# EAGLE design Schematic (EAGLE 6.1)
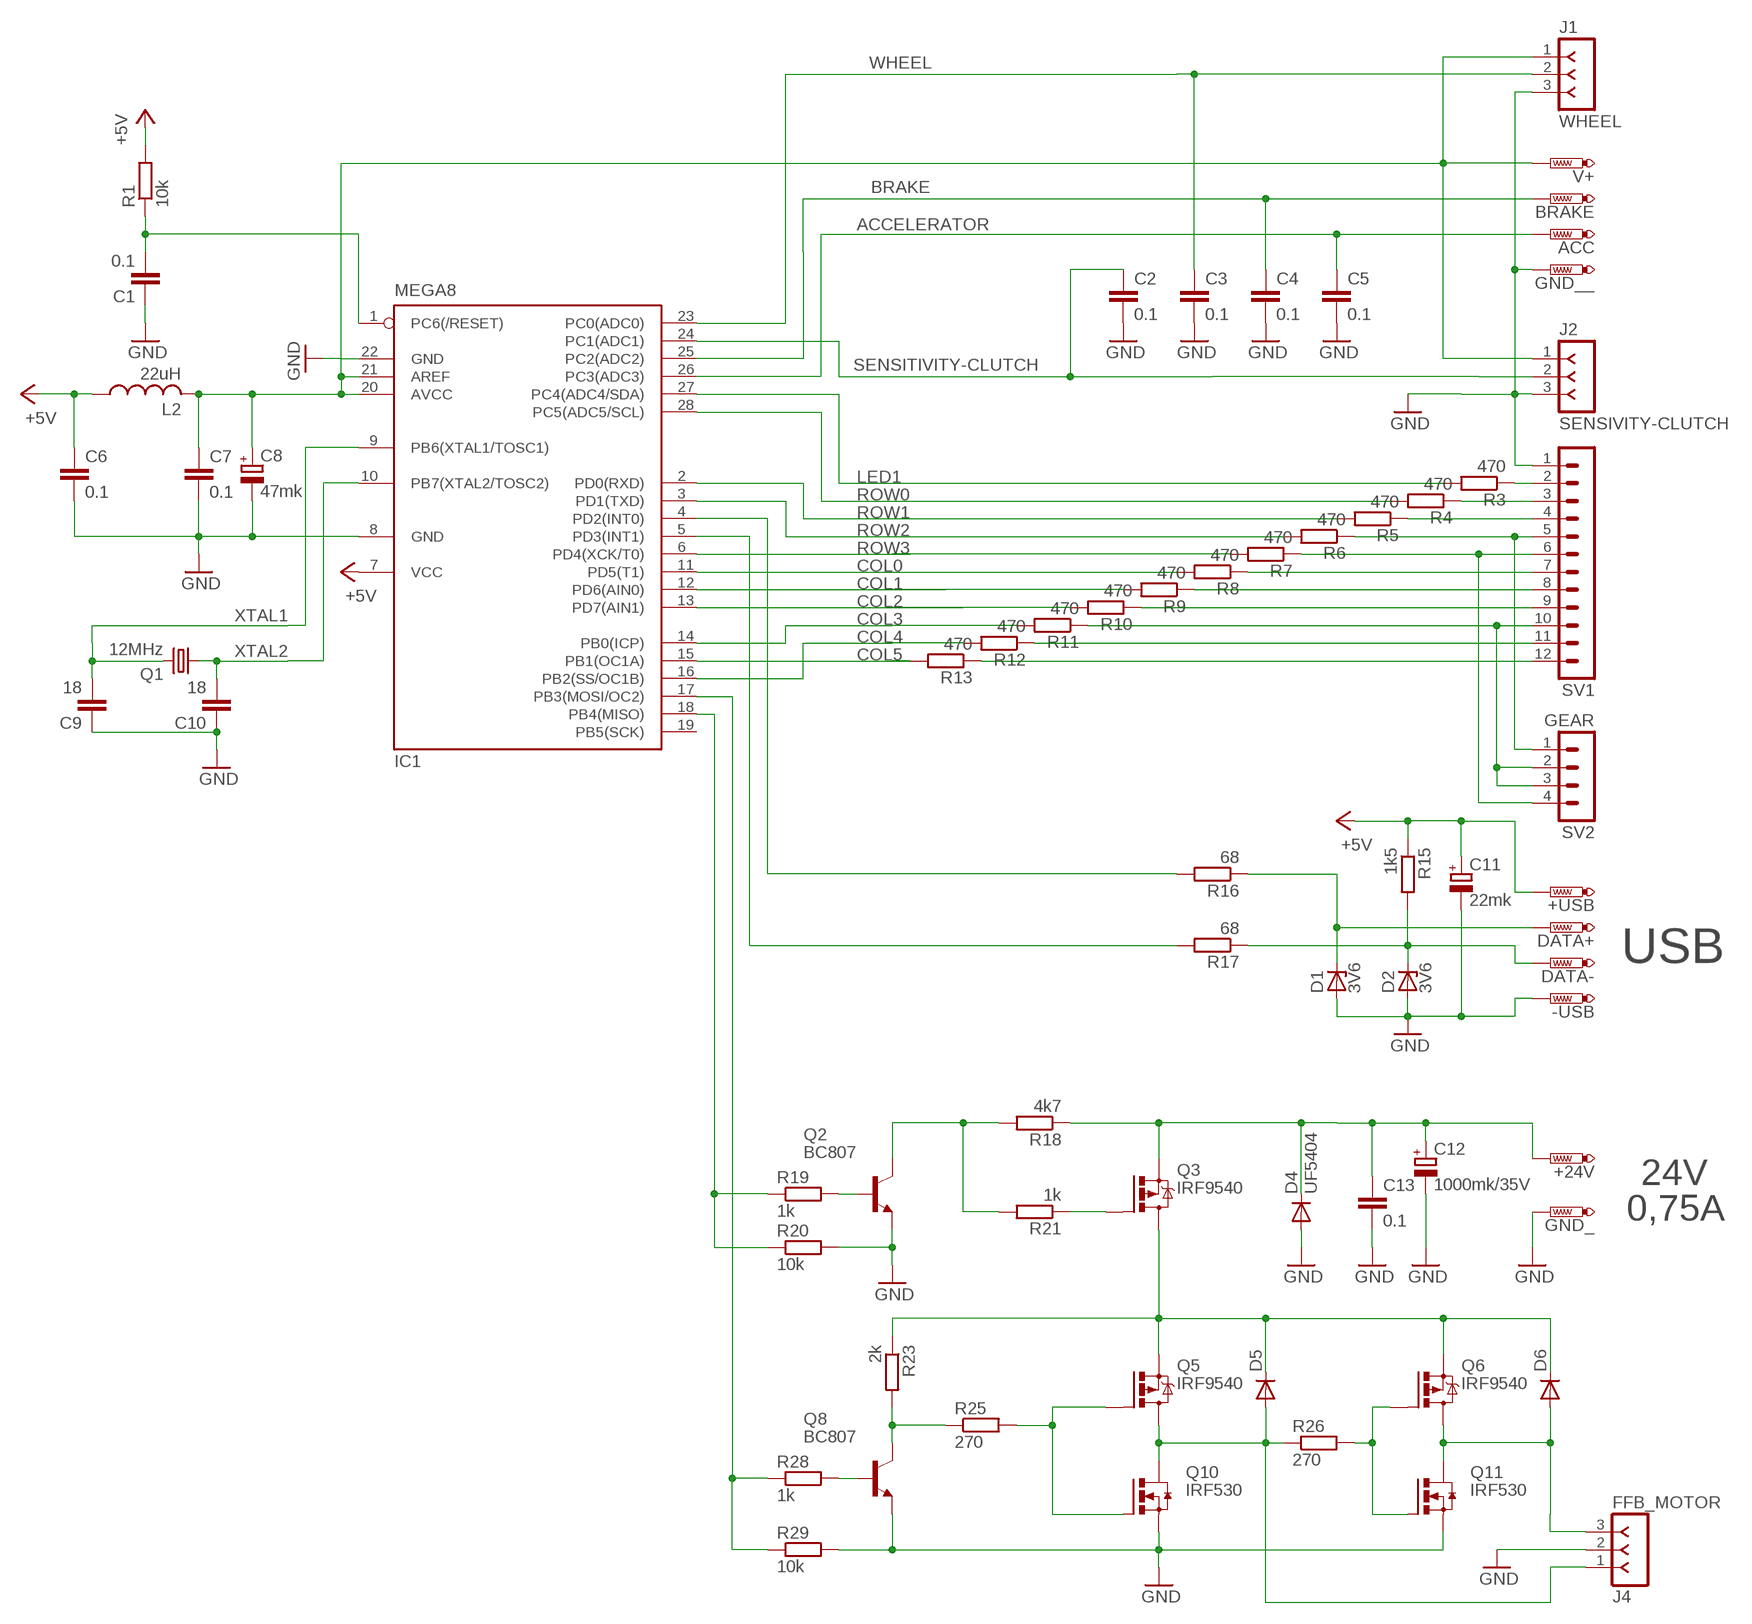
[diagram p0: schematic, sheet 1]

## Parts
+24V  PTR1PAD1-13  [P1-13]
+USB  PTR1PAD1-13  [P1-13]
-USB  PTR1PAD1-13  [P1-13]
ACC  PTR1PAD1-13  [P1-13]
BRAKE  PTR1PAD1-13  [P1-13]
C1  0.1  C-EUC0805  [C0805]
C2  0.1  C-EUC0805  [C0805]
C3  0.1  C-EUC0805  [C0805]
C4  0.1  C-EUC0805  [C0805]
C5  0.1  C-EUC0805  [C0805]
C6  0.1  C-EUC0805  [C0805]
C7  0.1  C-EUC0805  [C0805]
C8  47mk  CPOL-EUE2.5-6  [E2,5-6]
C9  18  C-EUC0805  [C0805]
C10  18  C-EUC0805  [C0805]
C11  22mk  CPOL-EUE2.5-6  [E2,5-6]
C12  1000mk/35V  CPOL-EUTT5D11L  [TT5D11L]
C13  0.1  C-EU075-032X103  [C075-032X103]
D1  3V6  BZX84CSMD  [TO236]
D2  3V6  BZX84CSMD  [TO236]
D4  UF5404  1N5400  [DO201-15]
D5  1N5400  [DO201-15]
D6  1N5400  [DO201-15]
DATA+  PTR1PAD1-13  [P1-13]
DATA-  PTR1PAD1-13  [P1-13]
GND_  PTR1PAD1-13  [P1-13]
GND__  PTR1PAD1-13  [P1-13]
IC1  MEGA8  MEGA8-P  [DIL28-3]
J1  WHEEL  F-1X03-SIP-100-32Y  [SIP-100-03-32Y]
J2  SENSIVITY-CLUTCH  F-1X03-SIP-100-32Y  [SIP-100-03-32Y]
J4  FFB_MOTOR  F-1X03-SIP-100-32Y  [SIP-100-03-32Y]
L2  22uH  L-USL3216C  [L3216C]
Q1  12MHz  CRYTALHC49U-V  [HC49U-V]
Q2  BC807  BC847SMD  [SOT23]
Q3  IRF9540  IRF4905  [TO220BH]
Q5  IRF9540  IRF4905  [TO220BH]
Q6  IRF9540  IRF4905  [TO220BH]
Q8  BC807  BC847SMD  [SOT23]
Q10  IRF530  IRFI540NPBF  [TO220BH]
Q11  IRF530  IRFI540NPBF  [TO220BH]
R1  10k  R-EU_R0805  [R0805]
R3  470  R-EU_R0805  [R0805]
R4  470  R-EU_R0805  [R0805]
R5  470  R-EU_R0805  [R0805]
R6  470  R-EU_R0805  [R0805]
R7  470  R-EU_R0805  [R0805]
R8  470  R-EU_R0805  [R0805]
R9  470  R-EU_R0805  [R0805]
R10  470  R-EU_R0805  [R0805]
R11  470  R-EU_R0805  [R0805]
R12  470  R-EU_R0805  [R0805]
R13  470  R-EU_R0805  [R0805]
R15  1k5  R-EU_R0805  [R0805]
R16  68  R-EU_0207/12  [0207/12]
R17  68  R-EU_0207/12  [0207/12]
R18  4k7  R-EU_R0805  [R0805]
R19  1k  R-EU_R0805  [R0805]
R20  10k  R-EU_R0805  [R0805]
R21  1k  R-EU_R0805  [R0805]
R23  2k  R-EU_R0805  [R0805]
R25  270  R-EU_R1206  [R1206]
R26  270  R-EU_R1206  [R1206]
R28  1k  R-EU_R0805  [R0805]
R29  10k  R-EU_R0805  [R0805]
SV1  MA12-1  [MA12-1]
SV2  GEAR  MA04-1  [MA04-1]
V+  PTR1PAD1-13  [P1-13]

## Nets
+5V: +USB.1(TP) C6.1 C11.+ IC1.7(VCC) L2.1 R1.2 R15.1
ACCELERATOR: ACC.1(TP) C5.1 IC1.26(PC3(ADC3))
BRAKE: BRAKE.1(TP) C4.1 IC1.25(PC2(ADC2))
COL0: IC1.11(PD5(T1)) R8.2
COL1: IC1.12(PD6(AIN0)) R9.2
COL2: IC1.13(PD7(AIN1)) R10.2
COL3: IC1.14(PB0(ICP)) R11.2
COL4: IC1.16(PB2(SS/OC1B)) R12.2
COL5: IC1.15(PB1(OC1A)) R13.2
FEEDBACK_MOTOR: IC1.17(PB3(MOSI/OC2)) R28.1 R29.1
GND: -USB.1(TP) C1.1 C2.2 C3.2 C4.2 C5.2 C6.2 C7.2 C8.- C9.1 C10.1 C11.- C12.- C13.2 D1.A D2.A D4.A GND_.1(TP) GND__.1(TP) IC1.8(GND) IC1.22(GND) J1.3 J2.3 J4.2 Q2.2(E) Q8.2(E) Q10.S Q11.S R20.2 R29.2 SV1.1
LED1: IC1.27(PC4(ADC4/SDA)) R3.2
M1: D5.A J4.1 Q5.D Q10.D R26.1
M2: D6.A J4.3 Q6.D Q11.D
N$1: D5.C D6.C Q3.D Q5.S Q6.S R23.1
N$2: C7.1 C8.+ IC1.20(AVCC) IC1.21(AREF) J1.1 J2.1 L2.2 V+.1(TP)
N$3: IC1.18(PB4(MISO)) R19.1 R20.1
N$4: +24V.1(TP) C12.+ C13.1 D4.C Q3.S R18.1
N$5: Q2.1(B) R19.2
N$6: IC1.5(PD3(INT1)) R17.2
N$8: IC1.4(PD2(INT0)) R16.2
N$9: D2.C DATA-.1(TP) R15.2 R17.1
N$10: D1.C DATA+.1(TP) R16.1
N$11: C1.2 IC1.1(PC6(/RESET)) R1.1
N$13: Q8.1(B) R28.2
N$14: Q8.3(C) R23.2 R25.1
N$15: R13.1 SV1.12
N$16: R11.1 SV1.10 SV2.2 SV2.3
N$19: Q5.G Q10.G R25.2
N$22: Q2.3(C) R18.2 R21.2
N$23: Q6.G Q11.G R26.2
N$30: R3.1 SV1.2
N$31: R4.1 SV1.3
N$32: R5.1 SV1.4
N$33: R6.1 SV1.5 SV2.1
N$34: R7.1 SV1.6 SV2.4
N$35: R8.1 SV1.7
N$36: R9.1 SV1.8
N$37: R10.1 SV1.9
N$39: R12.1 SV1.11
N$41: Q3.G R21.1
ROW0: IC1.28(PC5(ADC5/SCL)) R4.2
ROW1: IC1.2(PD0(RXD)) R5.2
ROW2: IC1.3(PD1(TXD)) R6.2
ROW3: IC1.6(PD4(XCK/T0)) R7.2
SENSITIVITY-CLUTCH: C2.1 IC1.24(PC1(ADC1)) J2.2
WHEEL: C3.1 IC1.23(PC0(ADC0)) J1.2
XTAL1: C9.2 IC1.9(PB6(XTAL1/TOSC1)) Q1.2
XTAL2: C10.2 IC1.10(PB7(XTAL2/TOSC2)) Q1.1
Unconnected: IC1.19(PB5(SCK))

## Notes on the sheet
- USB
- 24V
- 0,75A

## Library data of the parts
+24V +USB -USB ACC BRAKE DATA+ DATA- GND_ GND__ V+ = testpad:PTR1: TEST PIN
C1-C7 C9 C10 C13 = rcl:C-EU: CAPACITOR, European symbol
C8 C11 C12 = rcl:CPOL-EU: POLARIZED CAPACITOR, European symbol
D1 D2 = diode:BZX84CSMD: Z DIODE
D4-D6 = diode:1N5400: DIODE
IC1 = atmel:MEGA8-P: MICROCONTROLLER 8 Kbytes FLASH, 1 kbytes SRAM, 512 bytes EEPROM, USART, 4-channel 10 bit ADC, 2-channel 8 bit ADC Pin compatible with Atmega48, ATMega88, ATMega168 Source: avr.lbr; OC_FARNELL: unknown; OC_NEWARK: unknown
J1 J2 J4 = con-headers-jp:F-1X03-: FEMALE HEADER
L2 = rcl:L-US: INDUCTOR, American symbol
Q1 = crystal:CRYTAL: CRYSTAL
Q2 Q8 = transistor-npn:BC847*: NPN Transistor
Q3 Q5 Q6 = transistor-power:IRF4905: P-Channel HEXFET® Power MOSFET RDS(on)= 0.02 Ohm, ID = -74A Source: http://www.irf.com/product-info/datasheets/data/irf4905pbf.pdf
Q10 Q11 = transistor-power:IRFI540NPBF: HEXFET Power MOISFET VDSS = 100V, RDS(on) = 0.052 Ohm, ID = 20A, VGS(th) = 2.0 -- 4.0V Source: http://www.irf.com/product-info/datasheets/data/irfi540npbf.pdf
R1 R3-R13 R15-R21 R23 R25 R26 R28 R29 = rcl:R-EU_: RESISTOR, European symbol
SV1 = con-lstb:MA12-1: PIN HEADER; OC_FARNELL: unknown; OC_NEWARK: unknown
SV2 = con-lstb:MA04-1: PIN HEADER; OC_FARNELL: unknown; OC_NEWARK: unknown

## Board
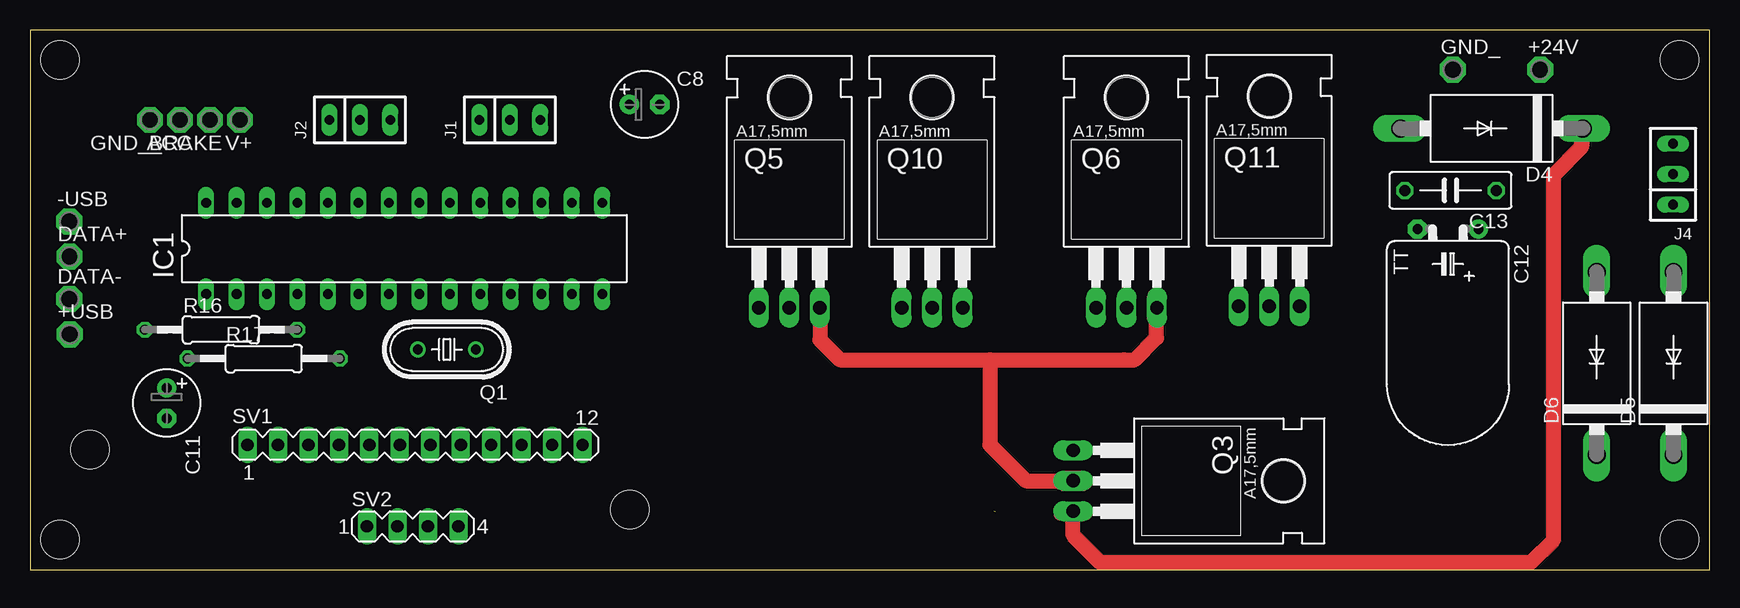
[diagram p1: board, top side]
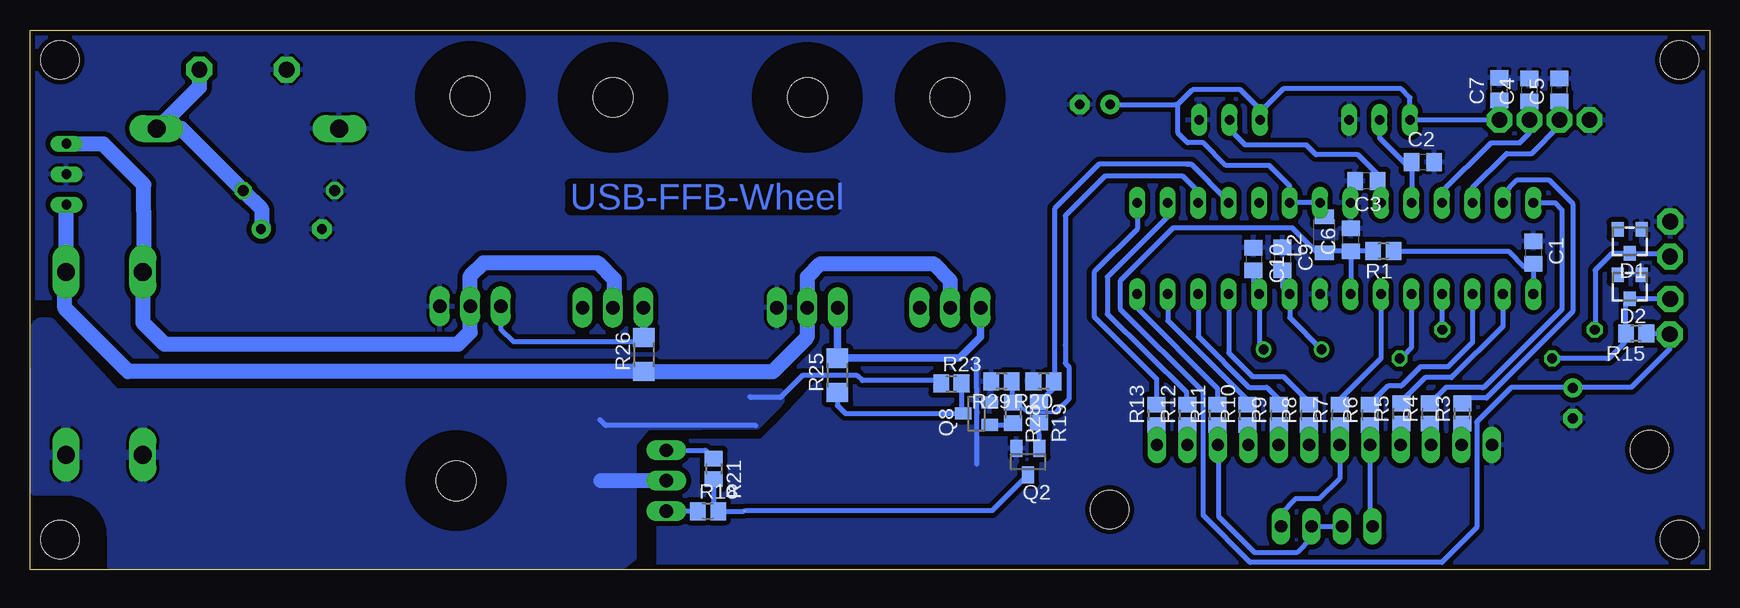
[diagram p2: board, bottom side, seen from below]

Size 140 x 45 mm. Coordinates in mm from the lower left corner, seen from the top.
Outline: 0,0 140,0 140,45 0,45 0,0
Copper layers (1*16): Top 0.035mm / dielectric 1.5mm / Bottom 0.035mm
Design rules: minimum track width 10mil, minimum drill 24mil, track to track 8mil, track to pad 8mil, pad to pad 8mil, via to via 8mil, smd to smd 8mil, copper to edge 1mil, drill to drill 8mil, minimum pad ring 10mil, minimum via ring 8mil, stop-mask expansion 4mil, vias tented up to drill 0mil, thermal gap 10mil
Holes 3.2 mm at 50,5 5,10 2.5,2.5 2.5,42.5 137.5,42.5 137.5,2.5

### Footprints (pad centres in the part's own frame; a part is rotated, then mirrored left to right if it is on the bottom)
P1-13 = drill 1.321 pad 2.159 octagon: 1 0,0
C0805 = smd 1.3 x 1.5: 1 -0.95,0; 2 0.95,0
E2,5-6 = drill 0.813 pad 1.6: + -1.27,0 | drill 0.813 pad 1.6 octagon: - 1.27,0
TT5D11L = drill 0.813 pad 1.6: + -2.54,0 | drill 0.813 pad 1.6 octagon: - 2.54,0
C075-032X103 = drill 0.914 octagon: 1 -3.81,0; 2 3.81,0
TO236 = smd 1 x 1.2: A -1,-1; C 0,1; NC 1,-1
DO201-15 = drill 1.499 long: A 7.62,0; C -7.62,0
DIL28-3 = drill 0.813 long: 1 -16.51,-3.81; 2 -13.97,-3.81; 3 -11.43,-3.81; 4 -8.89,-3.81; 5 -6.35,-3.81; 6 -3.81,-3.81; 7 -1.27,-3.81; 8 1.27,-3.81; 9 3.81,-3.81; 10 6.35,-3.81; 11 8.89,-3.81; 12 11.43,-3.81; 13 13.97,-3.81; 14 16.51,-3.81; 15 16.51,3.81; 16 13.97,3.81; 17 11.43,3.81; 18 8.89,3.81; 19 6.35,3.81; 20 3.81,3.81; 21 1.27,3.81; 22 -1.27,3.81; 23 -3.81,3.81; 24 -6.35,3.81; 25 -8.89,3.81; 26 -11.43,3.81; 27 -13.97,3.81; 28 -16.51,3.81
SIP-100-03-32Y = drill 0.813 long: 1 -2.54,0; 2 0,0; 3 2.54,0
L3216C = smd 1.2 x 1.6: 1 -1.5,0; 2 1.5,0
HC49U-V = drill 0.813: 1 -2.413,0; 2 2.413,0
SOT23 = smd 1 x 1.4: 1 -0.95,-1.1; 2 0.95,-1.1; 3 0,1.1
TO220BH = drill 1.118 long: D 0,-6.35; G -2.54,-6.35; S 2.54,-6.35 | hole 3.302: 0,11.176
R0805 = smd 1.3 x 1.5: 1 -0.85,0; 2 0.85,0
0207/12 = drill 0.813 octagon: 1 -6.35,0; 2 6.35,0
R1206 = smd 1.6 x 1.803: 1 -1.422,0; 2 1.422,0
MA12-1 = drill 1.016 long: 1 -13.97,0; 2 -11.43,0; 3 -8.89,0; 4 -6.35,0; 5 -3.81,0; 6 -1.27,0; 7 1.27,0; 8 3.81,0; 9 6.35,0; 10 8.89,0; 11 11.43,0; 12 13.97,0
MA04-1 = drill 1.016 long: 1 -3.81,0; 2 -1.27,0; 3 1.27,0; 4 3.81,0

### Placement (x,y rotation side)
+24V  125.88,41.7 0 top
+USB  3.32,19.62 0 top
-USB  3.27,29.02 0 top
ACC  12.5,37.5 180 top
BRAKE  15,37.5 180 top
C1  14.7,26.44 270 bottom
C2  23.9,34 0 bottom
C3  28.6,32.4 180 bottom
C4  15,40 90 bottom
C5  12.5,40 90 bottom
C6  29.9,27.5 90 bottom
C7  17.51,40.06 90 bottom
C8  51.23,38.79 0 top
C9  35.6,25.92 270 bottom
C10  38,25.9 270 bottom
C11  11.39,13.88 270 top
C12  118.2,28.4 180 top
C13  118.41,31.62 180 top
D1  6.65,27.37 180 bottom
D2  6.65,23.59 180 bottom
D4  121.83,36.79 180 top
D5  137,17.2 90 top
D6  130.6,17.2 90 top
DATA+  3.29,26.1 0 top
DATA-  3.27,22.56 0 top
GND_  118.6,41.7 0 top
GND__  10,37.5 180 top
IC1  31.19,26.78 0 top
J1  40,37.5 0 top
J2  27.5,37.5 0 top
J4  136.97,32.97 90 top
L2  32.1,27.93 90 bottom
Q1  34.75,18.35 180 top
Q2  56.8,9 180 bottom
Q3  93.3,7.4 270 top
Q5  63.3,28.2 0 top
Q6  91.4,28.2 0 top
Q8  61.1,13 90 bottom
Q10  75.2,28.2 0 top
Q11  103.3,28.3 0 top
R1  27.18,26.55 180 bottom
R3  20.6,13 90 bottom
R4  23.3,13 90 bottom
R5  25.7,13 90 bottom
R6  28.3,12.9 90 bottom
R7  30.8,12.9 90 bottom
R8  33.4,12.9 90 bottom
R9  35.9,12.9 90 bottom
R10  38.5,12.9 90 bottom
R11  41,12.9 90 bottom
R12  43.5,12.9 90 bottom
R13  46.1,12.9 90 bottom
R15  6.12,19.68 180 bottom
R16  15.92,20 0 top
R17  19.48,17.6 0 top
R18  83.49,4.87 0 bottom
R19  55.9,13.1 270 bottom
R20  55.5,15.7 180 bottom
R21  83,8.4 270 bottom
R23  63.2,15.5 0 bottom
R25  72.7,16.2 90 bottom
R26  88.82,17.94 90 bottom
R28  58.07,13.06 270 bottom
R29  59.01,15.7 180 bottom
SV1  32.1,10.4 0 top
SV2  31.9,3.6 0 top
V+  17.5,37.5 180 top

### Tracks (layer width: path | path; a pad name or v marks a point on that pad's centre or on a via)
+5V
  Bottom 0.406: R1.2 C6.1 | C6.1 | C6.1 29.9,22.99 IC1.7 | 11.5,15.2 6.5,15.2 3.32,18.38 +USB.1 3.4,19.7 3.5,19.7 3.52,19.68 R15.1 | 11.5,15.2 11.5,15.16 C11.+ | 11.5,15.2 16.5,15.2 19.4,12.3 19.4,3.5 22.3,0.6 38.3,0.6 42.2,4.5 42.2,14.8 49.1,21.7 49.1,24.1 44.7,28.52 34.8,28.52 32.73,26.43 L2.1 32.28,26.55 C6.1
ACCELERATOR
  Bottom 0.406: IC1.26 19.76,31.84 16.9,34.7 14.8,34.7 12.5,37 ACC.1 | ACC.1 | C5.1 ACC.1 | ACC.1 | ACC.1 12.5,37.6 | 12.5,37.6 | ACC.1 | ACC.1
BRAKE
  Bottom 0.406: IC1.25 22.3,31.5 18.2,35.6 15.8,35.6 15,36.4 BRAKE.1 | BRAKE.1 | C4.1 BRAKE.1 | BRAKE.1
COL0
  Bottom 0.406: IC1.11 40.08,18.08 38.1,16.1 35.5,16.1 33.3,13.9 33.4,13.8 R8.2
COL1
  Bottom 0.406: IC1.12 42.62,19.42 38.4,15.2 36.9,15.2 35.9,14.2 R9.2 | R9.2
COL2
  Bottom 0.406: IC1.13 45.16,20.76 38.4,14 38.4,13.85 R10.2
COL3
  Bottom 0.406: IC1.14 47.7,21.8 41,15.1 R11.2 | R11.2
COL4
  Bottom 0.406: IC1.16 45.16,29.44 50.2,24.4 50.2,21.3 43.6,14.8 43.6,13.85 R12.2
COL5
  Bottom 0.406: IC1.15 47.7,28.4 51.3,24.8 51.3,21.1 46.1,15.9 46.1,13.8 46.2,13.7 46.15,13.7 R13.2
FEEDBACK_MOTOR
  Bottom 0.305: 54.4,13.2 54.5,13.1 56.9,13.1 57.8,14
  Bottom 0.406: IC1.17 42.62,31.52 43.9,32.8 50.4,32.8 53.7,29.5 53.7,18.7 53.7,17.2 53.4,16.9 53.4,14.2 54.3,13.3 54.4,13.2 | 58.16,14.12 R28.1 57.98,14 57.8,14 | R29.1 58.16,14.12 | 58.16,14.12 58.16,14.1 | 58.16,14.1 58.16,14.06 58.1,14 | 58.16,14.12 58.16,14.1
GND
  Bottom 0.406: 61.1,17.4 61.1,15.1 61.1,10.2 61.1,8.8
  pour Bottom (isolate 0.406): 0,45 42.6,45 109.8,44.9 112.1,45.1 140,45 139.9,22.7 137.7,22.7 137.1,21.2 132,16.1 73.9,16.1 77.8,11.9 79,10.7 87.6,10.7 87.6,0.1 0,0
LED1
  Bottom 0.406: IC1.27 17.22,31.28 16,32.5 13.4,32.5 11.4,30.5 11.4,21.5 18.6,14.3 20.1,14.3 20.6,13.8 R3.2 | R3.2
M1
  Bottom 1.27: Q10.D 75.2,21.8 75.2,19.4 78.08,16.52 R26.1 131.82,16.52 137.1,21.8 137.1,24.72 D5.A 137,29.86 J4.1 | Q10.D | 75.2,21.9 75.2,24.4 74.1,25.5 64.7,25.5 63.3,24.1 63.3,21.5 | 63.3,21.5 63.4,21.4 | Q10.D 75.2,21.9 | 75.2,21.9 | Q5.D 63.3,21.5 | 63.3,21.5
M2
  Bottom 1.27: 103.3,21.8 103.3,19.8 104.3,18.8 128.8,18.8 130.6,20.6 D6.A 130.5,24.92 130.5,29.8 130.5,32.1 133.88,35.48 137.13,35.48 137.16,35.51 J4.3 | 103.3,21.8 Q11.D | Q11.D | 103.3,21.8 103.3,24.5 102.2,25.6 92.7,25.6 91.3,24.2 91.3,21.7 | 91.3,21.7 91.3,21.5 | Q6.D 91.4,21.8 91.3,21.7
N$1
  Top 1.27: 87.6,7.4 87.5,7.5 87.05,7.5 Q3.D | Q5.S 65.84,19.16 67.5,17.5 | 67.5,17.5 80,17.5 | 80,17.5 91.2,17.5 92.1,17.5 93.9,19.3 93.9,21.8 93.9,21.81 Q6.S | 67.5,17.5 80,17.5 | 80,17.5 80,10.4 83,7.4 Q3.D | Q3.D
  Bottom 0.406: R23.1 64.3,15.75 70.61,15.75 71.04,16.18 75.62,16.18 77.44,14.35 79.92,14.35 80,14.43 | 92,12 92.5,12.5 | 92.4,7.4 92.5,7.5 | 79.5,12 92,12 | 92,12 92.1,12.1
  Bottom 1.27: Q3.D 92.4,7.4
  pour Bottom: 133.2,0.4 90.7,0.4 89.8,1.1 89.8,10.5 88.6,12 79.4,12.1 77.7,13.8 77.7,13.9 77.5,14.1 77.5,14.7 132.9,14.7 138.3,20.6 139.2,20.6 139.5,20.3 139.6,6.6 136.8,6.6 arc90 133.2,2.6
N$2
  Bottom 0.406: V+.1 J2.1 | J2.1 | IC1.20 IC1.21 32.5,30.59 32.5,29.43 L2.2 | 37.4,38.1 37.4,38.5 37.6,38.5 39.1,40 43.1,40 44.3,38.8 | 37.4,38.1 37.4,37.56 J1.1 | IC1.20 35,32 36.7,33.7 40.3,33.7 42.2,35.6 43.5,35.6 44.3,36.4 44.3,38.8 | IC1.20 | J2.1 24.96,39.36 25.7,40.1 35.5,40.1 37.5,38.1 37.4,38.1 | C7.1 V+.1 | V+.1 | C8.+ 44.51,38.79 44.45,38.73 44.37,38.73 44.3,38.8
N$3
  Bottom 0.406: IC1.18 40.18,30.78 43.2,33.8 | 43.2,33.8 43.6,33.8 | 43.6,33.8 43.2,33.8 | 43.2,33.8 43.6,33.8 | 43.6,33.8 50.9,33.8 54.6,30.1 54.6,15.8 54.45,15.65 | 54.45,15.65 54.3,15.7 54.7,15.1 55.6,14.2 55.65,14.2 R19.1 | R20.1 54.5,15.6 54.45,15.65
N$4  (1 unrouted)
  Top 1.27: 127,32.8 127,2.5 125.1,0.6 89.2,0.6 86.94,2.86 Q3.S 86.9,4.9 86.91,4.9 Q3.S | 127,32.8 127,32.9 | 127,32.9 127,32.8 | 127,32.8 127,32.9 | 127,32.9 129.35,35.25 | 129.35,35.25 129.4,36.8 129.35,35.25
  Bottom 0.406: R18.1 Q3.S 86.16,4.86 86.3,5 | 129.3,36.8 129.8,36.8 129.3,36.8
  Bottom 1.016: 129.4,36.7 129.4,36.8 | 120.7,28.44 C12.+ 120.6,28.4 120.4,28.6 | C13.1
  Bottom 1.27: +24V.1 125.88,40.22 129.3,36.8 | 129.3,36.8 129.4,36.7 | 120.7,28.44 120.7,30.1 C13.1 127.39,36.79 D4.C 129.4,36.8 129.3,36.8
N$5
  Bottom 0.406: R19.2 55.9,11.3 55.9,10.1 | 55.9,10.1 | 55.9,10.1 Q2.1 | Q2.1
N$6
  Bottom 0.406: IC1.5 24.84,18.53 25.5,17.83 R17.2
N$8
  Bottom 0.305: 22.3,20 | 22.3,20 22.2,20 | R16.2 22.2,20 | 22.2,20
  Bottom 0.406: IC1.4 22.3,20
N$9
  Bottom 0.406: DATA-.1 3.3,22.59 D2.C 6.97,22.27 R15.2 6.97,19.13 7.1,19 7.1,18.9 8.4,17.6 8.55,17.6 R17.1 | R17.1
N$10
  Bottom 0.406: DATA+.1 3.56,26.37 D1.C 6.68,26.4 8.1,26.4 9.53,24.97 9.53,20.03 9.5,20 R16.1 | R16.1
N$11
  Bottom 0.406: 14.7,23 C1.2 14.3,25.1 14.8,25.6 15.39,25.19 16.7,26.5 26.28,26.5 R1.1 | 14.7,23 | 14.7,23 14.7,22.99 IC1.1
N$13
  Bottom 0.406: Q8.1 58.63,12.05 R28.2
N$14
  Bottom 0.406: R23.2 62.35,13.05 62.3,13 Q8.3 | 62.35,12.85 Q8.3 | Q8.3 | R25.1 72.7,13.67 72.03,13.01 Q8.3
N$15
  Bottom 0.406: R13.1 46.1,10.43 SV1.12
N$16
  Bottom 0.406: R11.1 SV1.10 40.9,10.31 40.9,4.4 37.9,1.4 34.4,1.4 33.17,2.63 SV2.3 SV2.2
N$19
  Bottom 0.406: 72.7,21.81 Q10.G
  Bottom 0.61: Q5.G 60.76,19.38 62.51,17.63 R25.2 72.7,21.81
N$21
  Top 0.305: 93.4,20.57 93.29,20.78 93.24,20.98 93.24,22.71 93.29,22.91 93.37,23.09 93.52,23.24 93.7,23.34 93.93,23.37 94.11,23.34 94.23,23.32 94.41,23.19 94.56,22.99 94.61,22.78 94.61,20.95 94.61,20.83 94.54,20.65 94.44,20.55 94.39,22.35 94.28,22.94 94.03,23.14 93.7,23.11 93.55,22.99 93.5,22.76 93.42,22.5 93.47,22.35 93.73,22.53 94.08,22.48 94.13,22.71 93.95,22.81 93.83,22.71 93.7,22.76 93.88,22.89 93.9,22.89
N$22  (1 unrouted)
  Bottom 0.406: R21.2 83,5.23 R18.2 80.48,4.87 | Q2.3 59.8,4.9 60.1,4.9 80.35,4.9
N$23
  Bottom 0.406: 88.8,21.91 Q6.G | Q11.G 100.76,20.06 99.7,19 88.9,19 88.8,18.9 88.8,19.34 R26.2
  Bottom 0.61: Q6.G 88.86,19.4 R26.2
N$24
  Top 0.305: 85.67,7.95 85.75,8 85.88,8.08 86.03,8.1 87.76,8.1 88.04,8.05 88.19,7.95 88.37,7.8 88.47,7.54 88.47,7.32 88.42,7.11 88.34,6.99 88.21,6.86 88.04,6.76 87.91,6.71 86.03,6.71 85.88,6.76 85.72,6.83 85.62,6.91 88.04,6.88 88.24,7.19 88.27,7.47 88.16,7.72 88.04,7.82
N$25
  Top 0.305: 86.39,4.22 86.31,4.17 86,4.19 85.8,4.24 85.62,4.37 85.47,4.57 85.42,4.83 85.45,5.08 85.6,5.31 85.78,5.46 85.98,5.54 87.86,5.54 88.01,5.51 88.16,5.44 88.34,5.28 88.44,5.11 88.49,4.9 88.47,4.72 88.42,4.55 88.34,4.42 88.21,4.29 88.04,4.22 87.88,4.19 87.83,4.17 87.61,4.17 87.61,5 87.38,5.33 87.86,5.33 88.09,5.21 88.21,4.9 88.09,4.6 87.76,4.42 88.29,4.62 87.83,4.9 87.76,5.13 87.99,5.03 87.86,4.67 86.28,4.42 85.88,4.45 85.67,4.67 85.7,4.93 85.85,5.21 86.13,5.31 86.46,5.31 86.21,5.11 86.23,4.88 86.26,4.67 86.03,4.65 85.85,4.72 86.08,4.88 86.08,4.95 85.95,4.95 86.06,5.03
N$26
  Top 0.305: 128.83,35.94 128.73,35.81 128.25,35.81 127.89,35.92 127.66,36.07 127.46,36.35 127.36,36.7 127.41,37.08 127.53,37.36 127.84,37.64 128.14,37.74 128.25,37.77 130.63,37.77 130.84,37.72 131.01,37.67 131.19,37.57 131.32,37.41 131.44,37.24 131.52,37.03 131.55,36.8 131.52,36.55 131.42,36.3 131.32,36.14 131.22,36.04 131.04,35.94 130.94,35.89 130.81,35.87 130.71,35.81 129.97,35.81 130.1,36.2 130.5,36.12 130.23,36.04 130.71,36.04 131.06,36.25 131.24,36.55 131.24,36.93 131.09,37.29 130.84,37.52 130.35,37.52 129.9,37.52 129.49,37.52 130,37.24 130.61,37.31 130.84,37.21 130.94,36.96 130.96,36.6 130.86,36.35 130.63,36.35 130.3,36.37 130.02,36.4 130.05,36.83 130.05,37.01 130.43,37.01 130.68,37.01 130.76,36.8 130.73,36.65 130.56,36.6 130.28,36.65 130.28,36.83 130.53,36.83 129.26,37.52 128.09,37.52 127.81,37.36 127.64,37.08 127.64,36.75 127.66,36.45 127.94,36.2 128.4,35.99 128.73,36.12 128.65,36.42 128.7,36.75 128.8,37.13 129.03,37.29 128.5,37.26 127.94,37.29 127.91,37.06 127.89,36.7 128.09,36.37 127.76,36.5 128.29,36.25 128.55,36.3 128.4,36.55 128.22,36.55 128.12,36.75 128.09,36.98 128.4,37.06 128.65,37.06 128.42,36.88 128.5,36.73 128.27,36.8
N$30
  Bottom 0.406: R3.1 20.6,10.4 | 20.6,10.4 | 20.6,10.4 SV1.2 | SV1.2
N$31
  Bottom 0.406: R4.1 23.3,10.49 SV1.3
N$32
  Bottom 0.406: R5.1 25.7,10.45 SV1.4
N$33
  Bottom 0.406: R6.1 SV1.5 | SV1.5 | SV1.5 28.3,3.61 SV2.1
N$34
  Bottom 0.406: R7.1 30.8,10.43 SV1.6 30.83,7.57 32.5,5.9 34.5,5.9 35.7,4.7 35.7,3.41 SV2.4
N$35
  Bottom 0.406: R8.1 33.4,10.43 SV1.7
N$36
  Bottom 0.406: R9.1 SV1.8
N$37
  Bottom 0.406: R10.1 38.5,10.45 SV1.9
N$39
  Bottom 0.406: R12.1 43.5,10.43 SV1.11
N$41
  Bottom 0.406: 83.04,9.22 R21.1 83.69,9.94 Q3.G
ROW0
  Bottom 0.406: IC1.28 12.89,30.59 12.3,30 12.3,21.7 18.8,15.2 | 18.8,15.2 19,15.2 18.8,15.2 | 18.8,15.2 21.95,15.2 R4.2
ROW1
  Bottom 0.406: IC1.2 17.22,20.28 21.5,16 23.7,16 25.9,13.8 25.65,13.8 R5.2 | 25.6,13.8 25.7,14 R5.2 | R5.2
ROW2
  Bottom 0.406: IC1.3 19.76,18.94 21.8,16.9 24.1,16.9 25.7,15.3 26.8,15.3 28.3,13.8 R6.2 | R6.2
ROW3
  Bottom 0.406: IC1.6 27.38,17.62 30.8,14.2 | R7.2 30.8,14.2 | 30.8,14.2
SENSITIVITY-CLUTCH
  Bottom 0.406: J2.2 | J2.2 27.5,36 24.8,33.3 | 24.8,33.3 24.8,34.1 | 24.8,34.1 24.8,33.3 | 24.8,33.3 24.8,30.63 IC1.24 | C2.1 24.85,34.05 24.8,34.1
WHEEL
  Bottom 0.406: IC1.23 27.38,32.68 | 27.38,32.68 29.3,34.6 32.8,34.6 33.6,35.4 38.7,35.4 39.6,36.3 J1.2 | J1.2 | 27.38,32.68 27.38,32.62 27.5,32.5 27.6,32.4 | 27.6,32.4 27.6,32.3 | C3.1 27.6,32.4 | 27.6,32.4
XTAL1
  Bottom 0.406: C9.2 35.6,23.57 IC1.9 35,21.01 Q1.2
XTAL2
  Bottom 0.406: C10.2 38,23.43 IC1.10 37.54,18.73 Q1.1

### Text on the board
Bottom: USB-FFB-Wheel
Document: Clutch | Wheel | C8 | Gnd | +24V | Gnd | Acc | Brake | V+ | 1 | 1 | D4 | Q5 | Q10 | Q6 | Q11 | C13 | Gnd | D+ | ATmega8 | D- | C12 | D6 | D5 | + | R16 | R17 | C11 | Buttons | Q3 | Gear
